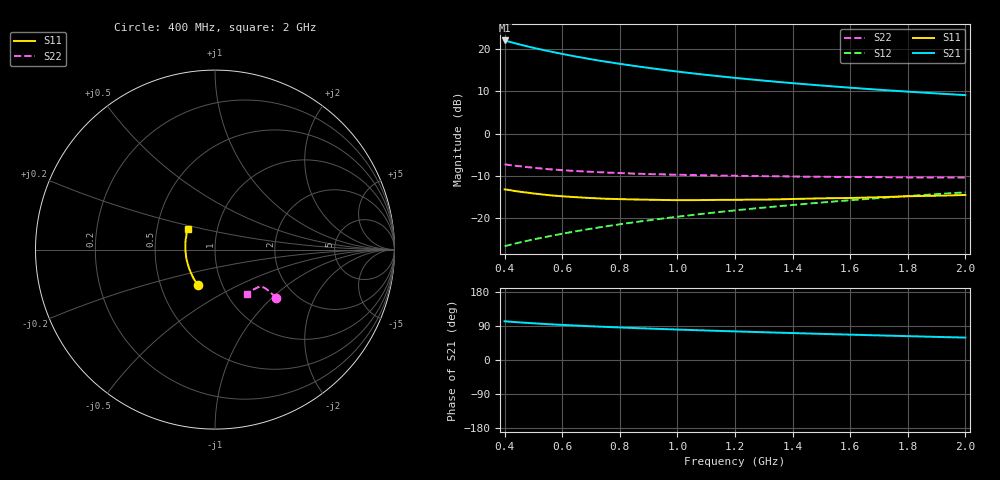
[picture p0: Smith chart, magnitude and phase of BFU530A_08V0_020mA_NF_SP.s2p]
! Filename:  P:\Prog\Test\Noise\ATS_data\Testdata_Net\06 Compressed Noise after Statistics\BFU530A_APG2013_33_A05_08p0V_020mA_NF_CM01_D.sf
! Date/Time: Tue 16/Apr/2013 15:10:58
! BFU530A_APG2013_33_A05_08p0V_1to25mA_NF_CM01_Bias7_R.sf
! Noise Parameter Data File
! BFU530A_APG2013_33_A05_08p0V_1to25mA_NF_CM01
! Date/time: Fri Apr 12 16:45:05 2013
! VAR V_out= 8.001000
! VAR I_out= 20.000000
! VAR V_in= 0.817300
! VAR I_in= 0.207350
! Device data file deembeded for feedlines and parallel
! Original file: \06 Compressed Noise after Statistics\BFU530A_APG2013_33_A05_08p0V_020mA_NF_CM01_R.sf
! Feed-files: PR017V01_150413_Feed1.s2p, PR017V01_150413_Feed2.s2p
! Parallel-file: PR017V01_150413_Par.s2p
# MHz S MA R 50
!  Freq-MHz  S11-mag  S11-arg  S21-mag  S21-arg  S12-mag  S12-arg  S22-mag  S22-arg
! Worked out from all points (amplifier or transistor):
!   37 points, 400 MHz to 2 GHz, reference 50 ohm
!   highest |S21| = 22.0 dB at 400 MHz (marker M1)
!   |S21| within 3 dB of that: start of sweep to 587.3 MHz
!   unconditionally stable (mu >= 1): 1.04 GHz to end of sweep
!   at 500 MHz: K = 0.92, MSG = 22.6 dB, |S12| = -25.0 dB
!   at 1.1 GHz: K = 1.00, MAG = 16.1 dB, |S12| = -18.8 dB
!   at 2 GHz: K = 1.00, MAG = 11.3 dB, |S12| = -13.8 dB
!   lowest NFmin = 1.06 dB at 433 MHz
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400  0.22 -115.3  12.53 102.2  0.04711 71.3  0.4342 -38.0
420  0.2151 -118.2  12 101.0  0.04901 71.4  0.4248 -38.0
433  0.2114 -120.0  11.69 100.3  0.0502 71.6  0.4195 -38.0
460  0.205 -123.3  11.06 98.8  0.05277 71.8  0.4096 -37.9
500  0.197 -128.4  10.26 96.9  0.05654 72.0  0.396 -37.8
550  0.1886 -134.4  9.423 94.6  0.06121 72.3  0.381 -37.6
600  0.1823 -139.5  8.691 92.6  0.06604 72.6  0.3707 -37.5
650  0.1779 -144.5  8.072 90.8  0.07084 72.7  0.362 -37.6
700  0.1739 -149.0  7.533 89.0  0.07566 72.8  0.3547 -37.6
750  0.1707 -153.4  7.06 87.4  0.08047 72.9  0.348 -37.7
800  0.1689 -157.4  6.648 85.9  0.08531 72.9  0.343 -38.0
850  0.1674 -161.5  6.28 84.4  0.09015 72.8  0.3377 -38.2
900  0.1662 -165.2  5.95 83.0  0.09504 72.8  0.3336 -38.5
950  0.1651 -168.7  5.655 81.7  0.09989 72.7  0.3305 -39.0
1050  0.1644 -175.0  5.145 79.1  0.1097 72.4  0.3247 -39.8
1150  0.1655 178.9  4.723 76.7  0.1195 72.0  0.3197 -40.8
1200  0.1657 176.3  4.539 75.5  0.1244 71.8  0.3183 -41.4
1350  0.1679 168.5  4.066 72.2  0.1392 71.0  0.314 -43.4
1500  0.1726 161.5  3.688 69.0  0.154 70.1  0.3096 -45.6
1650  0.176 155.6  3.38 65.9  0.1688 69.0  0.3075 -48.0
1750  0.1801 151.7  3.203 63.9  0.1786 68.3  0.3057 -49.7
2000  0.1892 143.6  2.841 59.1  0.2032 66.5  0.3034 -54.4
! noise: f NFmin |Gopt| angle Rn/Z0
400  1.103  0.2145  -168.4  0.0889
460  1.057  0.2193  -167.3  0.0874
600  1.141  0.2153  -159.8  0.0982
800  1.107  0.2392  -159.7  0.0888
1000  1.14  0.2588  -155  0.0856
1200  1.163  0.2666  -146.5  0.0979
1400  1.212  0.2837  -143.1  0.0975
1600  1.211  0.3013  -137.8  0.0995
1800  1.177  0.3371  -133.4  0.1034
2000  1.214  0.354  -129.1  0.1091
